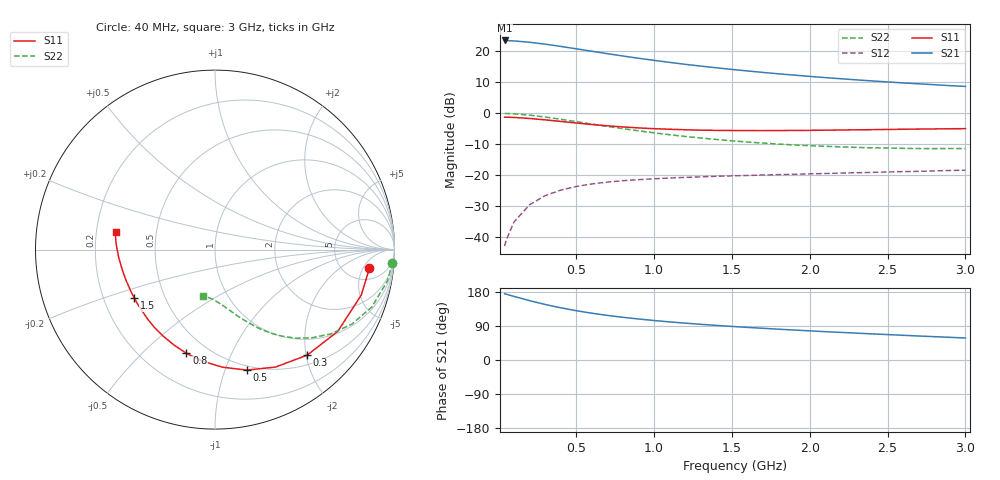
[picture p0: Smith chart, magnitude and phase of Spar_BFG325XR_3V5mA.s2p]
! Filename: 35BFG325XR.s2p
! Title: BFG325XR,RN20042071,Lot:TT3899C,B:Y13641,Sl.:1
! Bias: VCE=2.999V; IC=4.957mA;
! Company: NXP Semiconductors NL
! User: Q&R DSC-N
! Measure time: 29 Mar 2004 / 13:38:35
#  MHz  S  MA  R 50
! Freq  S11  S21  S12  S22  :
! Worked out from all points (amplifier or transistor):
!   32 points, 40 MHz to 3 GHz, reference 50 ohm
!   highest |S21| = 23.5 dB at 40 MHz (marker M1)
!   |S21| within 3 dB of that: start of sweep to 538.5 MHz
!   unconditionally stable (mu >= 1): 2.979 GHz to end of sweep
!   at 400 MHz: K = 0.23, MSG = 23.2 dB, |S12| = -24.9 dB
!   at 1.5 GHz: K = 0.70, MSG = 17.2 dB, |S12| = -20.3 dB
!   at 3 GHz: K = 1.00, MAG = 13.2 dB, |S12| = -18.4 dB
!   S11 on the Smith chart (normalised r, x): 40 MHz: 8, -7; 300 MHz: 0.67, -2.02; 500 MHz: 0.46, -1.19; 800 MHz: 0.38, -0.69; 1.5 GHz: 0.33, -0.25; 3 GHz: 0.28, +0.08
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40  0.8628 -6.9  14.98 174.9  0.007094 86.0  0.9905 -4.2
50  0.8623 -8.7  14.93 173.7  0.008836 85.0  0.9888 -5.2
100  0.8534 -17.3  14.72 167.9  0.0174 80.2  0.9761 -10.4
200  0.8219 -33.7  14 156.7  0.03313 71.5  0.9309 -20.1
300  0.7807 -48.9  13.06 146.6  0.04644 63.8  0.8679 -28.6
400  0.7362 -62.7  12.01 137.8  0.05706 57.3  0.798 -36.0
500  0.6944 -75.2  10.98 130.1  0.06543 52.2  0.73 -42.3
600  0.6563 -86.4  10.03 123.5  0.07188 47.9  0.6676 -47.6
700  0.6253 -96.4  9.167 117.7  0.07696 44.5  0.6112 -52.2
800  0.5996 -105.4  8.394 112.7  0.08111 41.8  0.5619 -56.1
900  0.5782 -113.5  7.724 108.2  0.08434 39.7  0.5191 -59.5
1000  0.5617 -121.0  7.14 104.2  0.08712 38.0  0.4821 -62.5
1100  0.5501 -127.6  6.624 100.5  0.08963 36.6  0.4487 -65.3
1200  0.5399 -133.7  6.166 97.3  0.09168 35.6  0.4205 -68.0
1300  0.5316 -139.2  5.766 94.1  0.09367 34.7  0.3971 -70.6
1500  0.5248 -149.0  5.094 88.6  0.09705 33.7  0.3577 -75.0
1600  0.5231 -153.3  4.816 86.0  0.09858 33.1  0.3417 -77.3
1800  0.5245 -161.0  4.323 81.3  0.1016 32.8  0.317 -81.5
2100  0.5312 -170.5  3.756 74.8  0.106 32.6  0.2917 -87.7
2300  0.5387 -175.6  3.455 70.9  0.1091 32.8  0.2796 -91.4
2600  0.55 177.6  3.083 65.2  0.1136 33.2  0.2702 -97.1
3000  0.5625 170.2  2.708 58.0  0.1201 33.4  0.2679 -104.1
